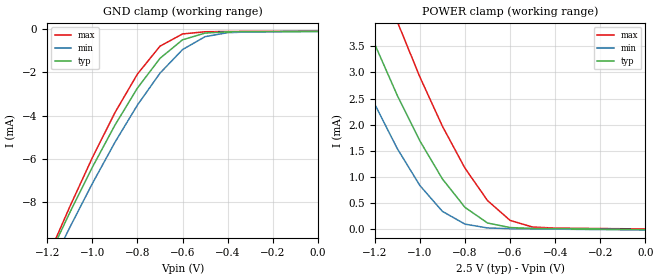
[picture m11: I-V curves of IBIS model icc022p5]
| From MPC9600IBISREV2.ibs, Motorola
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|This is a Model of an Input with a 25,000 ohm Pull_up at 2.5V
[Model]   icc022p5
Model_type   Input
Vmeas=1.25
Vinl=.7
Vinh=1.7
| Variable   typ   min   max
C_comp   5p   5p   5p
[Temperature Range]   27.00   100.00   -45.00
[Power Clamp Reference]   2.50V   2.25V   2.75V
[Gnd Clamp Reference]   0.000V   0.000V   0.000V
[Voltage Range]   2.50V   2.25V   2.75V
[Pulldown Reference]   0.000V   0.000V   0.000V
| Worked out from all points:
|   GND clamp passes 1 mA (typ) near -0.66 V on its own axis
|   POWER clamp passes 1 mA (typ) near -0.90 V on its own axis
[GND_clamp]
| voltage   I(typ)   I(min)   I(max)
-2.5V     -42.51mA   -42.15mA   -44.31mA
-1.2V     -10.71mA   -11.32mA   -10.62mA
-1.1V     -8.502mA   -9.191mA   -8.23mA
-1V       -6.399mA   -7.155mA   -5.958mA
-900mV    -4.45mA    -5.246mA   -3.87mA
-800mV    -2.726mA   -3.513mA   -2.077mA
-700mV    -1.348mA   -2.036mA   -784.8uA
-600mV    -489.4uA   -942.6uA   -218uA
-500mV    -177.2uA   -344uA     -117uA
-400mV    -120.2uA   -158.5uA   -105.2uA
1.08fV    -99.01uA   -108.9uA   -89.1uA
[POWER_clamp]
| voltage   I(typ)  I(min)  I(max)
-2.5V     21.02mA    19.16mA    23.53mA
-1.4V     5.76mA     4.398mA    7.621mA
-1.3V     4.611mA    3.352mA    6.339mA
-1.2V     3.54mA     2.394mA    5.117mA
-1.1V     2.561mA    1.545mA    3.97mA
-1V       1.694mA    841.2uA    2.915mA
-900mV    965.7uA    346.2uA    1.972mA
-800mV    422.8uA    102.4uA    1.172mA
-700mV    124uA      28.88uA    552.3uA
-600mV    35.95uA    15.08uA    173.7uA
-500mV    20.84uA    10.02uA    45.83uA
1.08fV    26.02pA    -9.897uA   9.901uA
